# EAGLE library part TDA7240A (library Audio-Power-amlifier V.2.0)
The TDA7240A is a 20W bridge audio amplifier IC designed specially for car radio applications. Thanks to the low external part count and compact Heptawatt 7-pin power package the TDA7240A occupies little space on the printed circuit board.
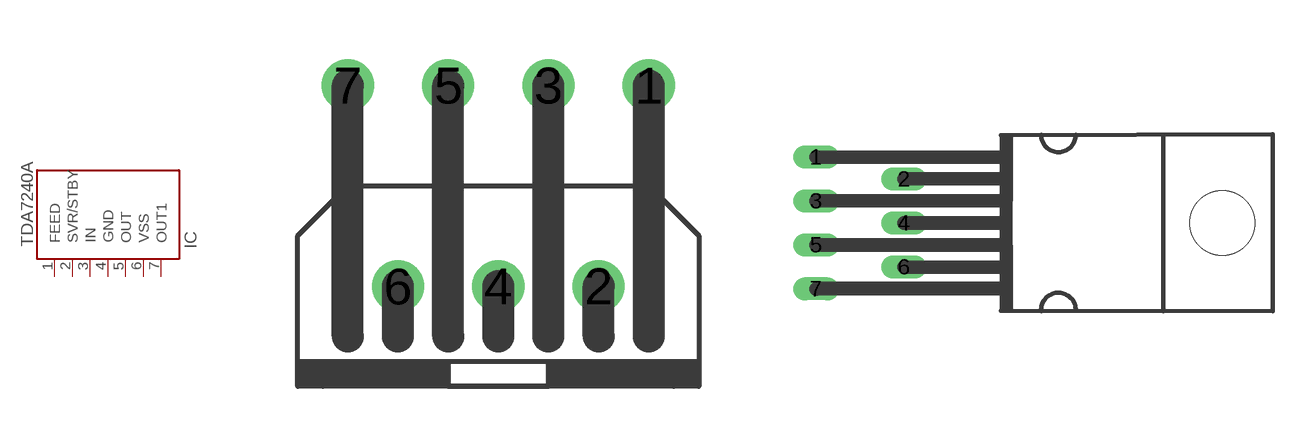
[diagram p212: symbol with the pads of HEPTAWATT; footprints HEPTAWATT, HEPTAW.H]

Designator prefix IC

## TDA7240ATDA7240AV  [HEPTAWATT]
1  FEED
2  SVR/STBY
3  IN
4  GND  pwr
5  OUT  out
6  VSS  pwr
7  OUT1  out

## TDA7240ATDA7240AH  [HEPTAW.H]
Pads as for HEPTAWATT

## Footprint HEPTAWATT (pad centres in mm)
HEPTAWATT 7
drill 0.813: 1 3.81,5.08; 2 2.54,0; 3 1.27,5.08; 4 0,0; 5 -1.27,5.08; 6 -2.54,0; 7 -3.81,5.08

## Footprint HEPTAW.H (pad centres in mm)
drill 0.813 long: 1 -11.43,3.81; 2 -6.35,2.54; 3 -11.43,1.27; 4 -6.35,0; 5 -11.43,-1.27; 6 -6.35,-2.54; 7 -11.43,-3.81
hole 3.75 at 12.05,0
